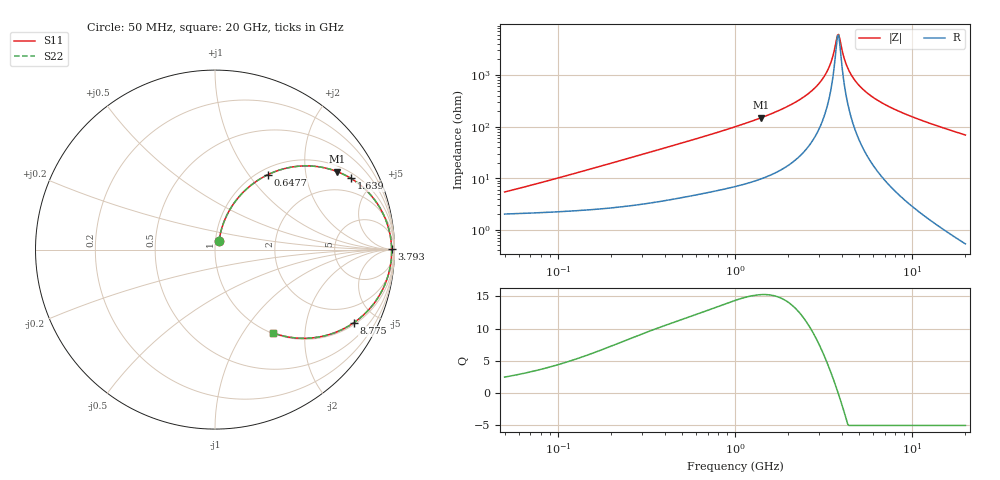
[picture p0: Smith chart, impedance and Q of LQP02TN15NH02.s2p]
!Murata Part Number: LQP02TN15NH02
!These Parameters are Measured in Series Mode Connection
!  o--[Z]--o
!Port1  Port2
!  o-------o
!Freq. Start=50[MHz] Stop=20[GHz], 401[Steps]
# Hz S RI R 50
!Freq.(Hz) S11(Real) S11(Imag) S21(Real) S21(Imag) S12(Real) S12(Imag) S22(Real) S22(Imag)
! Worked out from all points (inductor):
!   401 points, 50 MHz to 20 GHz, reference 50 ohm
!   read as one part in series: L = 15.8 nH near 62.6 MHz
!   highest Q = 15.3 at 1.411 GHz (marker M1), where L = 16.8 nH
!   self-resonance near 3.793 GHz
!   S11 on the Smith chart (normalised r, x): 50 MHz: 1.04, +0.10; 647.7 MHz: 1.10, +1.25; 1.639 GHz: 1.24, +3.66; 3.793 GHz: open; 8.775 GHz: 1.08, -3.73; 20 GHz: 1.01, -1.38
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5e7  0.0223 0.0482  0.9777 -0.0482  0.9777 -0.0482  0.0223 0.0482
1.364002e8  0.0397 0.1252  0.9603 -0.1252  0.9603 -0.1252  0.0397 0.1252
3.721004e8  0.137 0.298  0.863 -0.298  0.863 -0.298  0.137 0.298
6.476653e8  0.2954 0.4179  0.7046 -0.4179  0.7046 -0.4179  0.2954 0.4179
1e9  0.4958 0.4663  0.5042 -0.4663  0.5042 -0.4663  0.4958 0.4663
1.411297e9  0.6802 0.4348  0.3198 -0.4348  0.3198 -0.4348  0.6802 0.4348
1.639343e9  0.7565 0.3974  0.2435 -0.3974  0.2435 -0.3974  0.7565 0.3974
2.179053e9  0.8784 0.2912  0.1216 -0.2912  0.1216 -0.2912  0.8784 0.2912
2.728004e9  0.9443 0.1831  0.0557 -0.1831  0.0557 -0.1831  0.9443 0.1831
3.029571e9  0.9645 0.128  0.0355 -0.128  0.0355 -0.128  0.9645 0.128
3.314454e9  0.9762 0.0793  0.0238 -0.0793  0.0238 -0.0793  0.9762 0.0793
3.519108e9  0.9812 0.0463  0.0188 -0.0463  0.0188 -0.0463  0.9812 0.0463
3.792786e9  0.9841 0.0047  0.0159 -0.0047  0.0159 -0.0047  0.9841 0.0047
3.908127e9  0.9843 -0.012  0.0157 0.012  0.0157 0.012  0.9843 -0.012
4.149438e9  0.9828 -0.0454  0.0172 0.0454  0.0172 0.0454  0.9828 -0.0454
4.34015e9  0.9802 -0.0705  0.0198 0.0705  0.0198 0.0705  0.9802 -0.0705
4.81993e9  0.969 -0.1284  0.031 0.1284  0.031 0.1284  0.969 -0.1284
5.769027e9  0.933 -0.2243  0.067 0.2243  0.067 0.2243  0.933 -0.2243
7.442007e9  0.847 -0.3452  0.153 0.3452  0.153 0.3452  0.847 -0.3452
8.774992e9  0.7718 -0.4086  0.2282 0.4086  0.2282 0.4086  0.7718 -0.4086
1.295331e10  0.5565 -0.4904  0.4435 0.4904  0.4435 0.4904  0.5565 -0.4904
2e10  0.3228 -0.4637  0.6772 0.4637  0.6772 0.4637  0.3228 -0.4637
